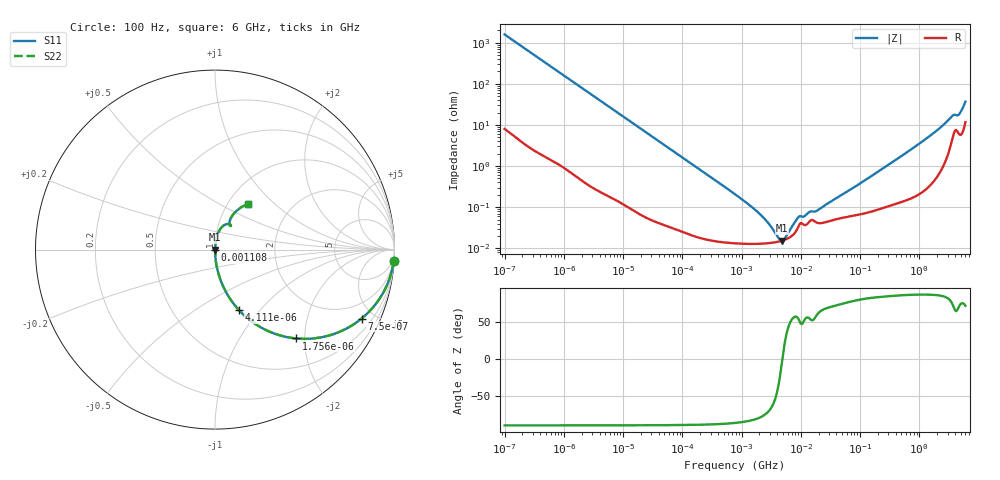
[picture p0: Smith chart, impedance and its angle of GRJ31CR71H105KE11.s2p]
!Murata Part Number: GRJ31CR71H105KE11
!These Parameters are Measured in Series Mode Connection
!Data Generated on Jun 19, 2026
!  o--ll--o
!Port1  Port2
!  o------o
!Operation Temp=25[degC], DC Bias Voltage=0[V]
!Freq. Start=100[Hz] Stop=6[GHz] 401[Steps]
# Hz S RI R 50
!Freq.(Hz) S11(Real) S11(Imag) S21(Real) S21(Imag) S12(Real) S12(Imag) S22(Real) S22(Imag)
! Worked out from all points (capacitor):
!   401 points, 100 Hz to 6 GHz, reference 50 ohm
!   read as one part in series: C = 1.01 uF near 109 Hz
!   lowest |Z| = 15.3 mohm at 4.857 MHz (marker M1)
!   series resonance near 4.886 MHz, so ESL is about 1.1 nH
!   S11 on the Smith chart (normalised r, x): 100 Hz: 1, -32; 750 Hz: 1.02, -4.24; 1.756 kHz: 1.01, -1.82; 4.111 kHz: 1.00, -0.78; 1.108 MHz: 1.00, -0.00; 6 GHz: 1.23, +0.70
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100  0.9957 -0.063  0.0043 0.063  0.0043 0.063  0.9957 -0.063
350  0.9526 -0.2102  0.0474 0.2102  0.0474 0.2102  0.9526 -0.2102
750  0.8167 -0.3842  0.1833 0.3842  0.1833 0.3842  0.8167 -0.3842
1756  0.4524 -0.495  0.5476 0.495  0.5476 0.495  0.4524 -0.495
2008  0.3877 -0.4845  0.6123 0.4845  0.6123 0.4845  0.3877 -0.4845
4111  0.1329 -0.3365  0.8671 0.3365  0.8671 0.3365  0.1329 -0.3365
11514  0.0201 -0.1366  0.9799 0.1366  0.9799 0.1366  0.0201 -0.1366
40335  0.002 -0.0399  0.998 0.0399  0.998 0.0399  0.002 -0.0399
774597  0.000136 -0.00206  0.9999 0.00206  0.9999 0.00206  0.000136 -0.00206
1108252  0.00013 -0.0014  0.9999 0.0014  0.9999 0.0014  0.00013 -0.0014
2268635  0.00013 -0.000568  0.9999 0.000568  0.9999 0.000568  0.00013 -0.000568
4246196  0.000146 -9.55e-05  0.9999 9.55e-05  0.9999 9.55e-05  0.000146 -9.55e-05
4856642  0.000153 -4e-06  0.9998 4e-06  0.9998 4e-06  0.000153 -4e-06
5554849  0.000164 8.85e-05  0.9998 -8.85e-05  0.9998 -8.85e-05  0.000164 8.85e-05
9090158  0.000336 0.000461  0.9997 -0.000461  0.9997 -0.000461  0.000336 0.000461
1.555665e7  0.000487 0.000618  0.9995 -0.000618  0.9995 -0.000618  0.000487 0.000618
1.946e7  0.000412 0.000741  0.9996 -0.000741  0.9996 -0.000741  0.000412 0.000741
3.124326e8  0.00119 0.011  0.9988 -0.011  0.9988 -0.011  0.00119 0.011
1.497423e9  0.00609 0.0529  0.9939 -0.0529  0.9939 -0.0529  0.00609 0.0529
3.505958e9  0.0578 0.1399  0.9422 -0.1399  0.9422 -0.1399  0.0578 0.1399
4.586474e9  0.0806 0.1414  0.9194 -0.1414  0.9194 -0.1414  0.0806 0.1414
6e9  0.1845 0.2556  0.8155 -0.2556  0.8155 -0.2556  0.1845 0.2556
